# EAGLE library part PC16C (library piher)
POTENTIOMETER quad carbon potentiometer, 16 mm
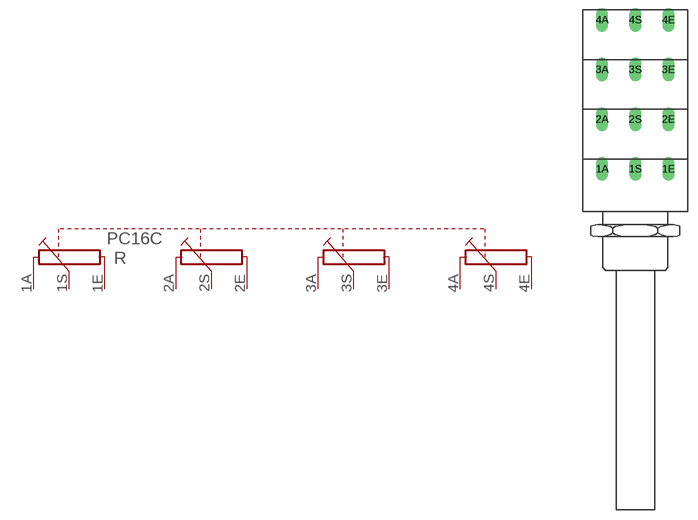
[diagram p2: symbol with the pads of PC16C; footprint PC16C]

Designator prefix R

## PC16C (OC_FARNELL: 3605360; OC_NEWARK: unknown)  [PC16C]
1A  1A  pas
1E  1E  pas
1S  1S  pas
2A  2A  pas
2E  2E  pas
2S  2S  pas
3A  3A  pas
3E  3E  pas
3S  3S  pas
4A  4A  pas
4E  4E  pas
4S  4S  pas

## Footprint PC16C (pad centres in mm)
POTENTIOMETER quad carbon potentiometer, 16 mm
drill 1.2 long: 1A -5,6.5; 1E 5,6.5; 1S 0,6.5; 2A -5,14; 2E 5,14; 2S 0,14; 3A -5,21.5; 3E 5,21.5; 3S 0,21.5; 4A -5,29; 4E 5,29; 4S 0,29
